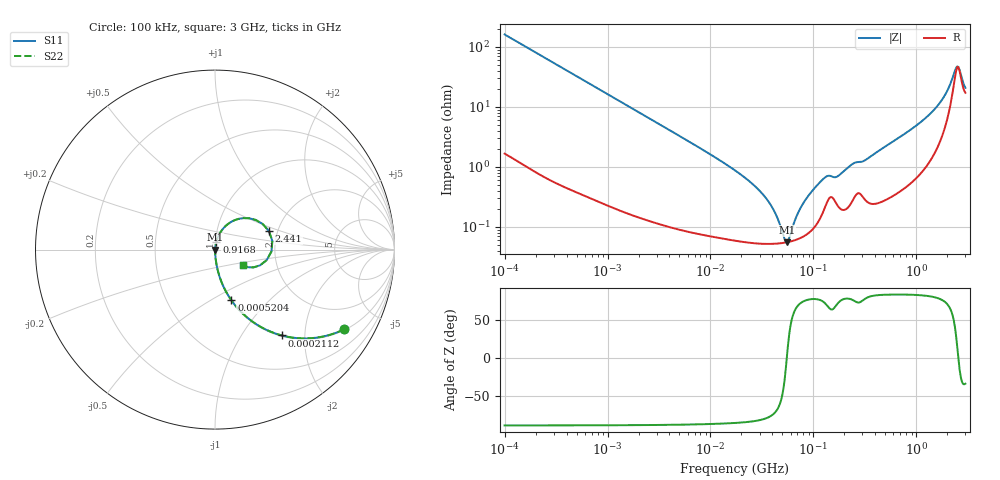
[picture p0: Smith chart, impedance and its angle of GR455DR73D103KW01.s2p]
!Murata Part Number: GR455DR73D103KW01
!These Parameters are Measured in Series Mode Connection
!Data Generated on Mar 13, 2026
!  o--ll--o
!Port1  Port2
!  o------o
!Operation Temp=25[degC], DC Bias Voltage=0[V]
!Freq. Start=100[kHz] Stop=3[GHz] 401[Steps]
# Hz S RI R 50
!Freq.(Hz) S11(Real) S11(Imag) S21(Real) S21(Imag) S12(Real) S12(Imag) S22(Real) S22(Imag)
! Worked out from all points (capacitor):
!   401 points, 100 kHz to 3 GHz, reference 50 ohm
!   read as one part in series: C = 9.88 nF near 105.3 kHz
!   lowest |Z| = 55.4 mohm at 55.24 MHz (marker M1)
!   series resonance near 55.22 MHz, so ESL is about 840 pH
!   S11 on the Smith chart (normalised r, x): 100 kHz: 1.03, -3.22; 211.2 kHz: 1.02, -1.53; 520.4 kHz: 1.01, -0.62; 916.8 MHz: 1.01, +0.09; 2.441 GHz: 1.80, +0.41; 3 GHz: 1.34, -0.23
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100000  0.7191 -0.4443  0.2809 0.4443  0.2809 0.4443  0.7191 -0.4443
211150  0.3707 -0.478  0.6293 0.478  0.6293 0.478  0.3707 -0.478
520403  0.0915 -0.2825  0.9085 0.2825  0.9085 0.2825  0.0915 -0.2825
562235  0.0798 -0.265  0.9202 0.265  0.9202 0.265  0.0798 -0.265
3161081  0.00379 -0.0516  0.9962 0.0516  0.9962 0.0516  0.00379 -0.0516
1.77727e7  0.000656 -0.00845  0.9993 0.00845  0.9993 0.00845  0.000656 -0.00845
3.564176e7  0.000528 -0.00277  0.9995 0.00277  0.9995 0.00277  0.000528 -0.00277
4.268829e7  0.000527 -0.0016  0.9995 0.0016  0.9995 0.0016  0.000527 -0.0016
5.246276e7  0.000545 -0.000317  0.9995 0.000317  0.9995 0.000317  0.000545 -0.000317
5.523785e7  0.000554 2.3e-06  0.9994 -2.3e-06  0.9994 -2.3e-06  0.000554 2.3e-06
7.334282e7  0.000645 0.00181  0.9994 -0.00181  0.9994 -0.00181  0.000645 0.00181
9.738194e7  0.00091 0.00386  0.9991 -0.00386  0.9991 -0.00386  0.00091 0.00386
1.326759e8  0.00237 0.00641  0.9976 -0.00641  0.9976 -0.00641  0.00237 0.00641
1.716802e8  0.00231 0.00654  0.9977 -0.00654  0.9977 -0.00654  0.00231 0.00654
2.400085e8  0.00283 0.0108  0.9972 -0.0108  0.9972 -0.0108  0.00283 0.0108
5.475153e8  0.00358 0.0238  0.9964 -0.0238  0.9964 -0.0238  0.00358 0.0238
9.167529e8  0.00745 0.0428  0.9926 -0.0428  0.9926 -0.0428  0.00745 0.0428
1.838476e9  0.0534 0.1259  0.9466 -0.1259  0.9466 -0.1259  0.0534 0.1259
2.201951e9  0.1571 0.1754  0.8429 -0.1754  0.8429 -0.1754  0.1571 0.1754
2.441062e9  0.3004 0.1031  0.6996 -0.1031  0.6996 -0.1031  0.3004 0.1031
2.706139e9  0.2511 -0.0875  0.7489 0.0875  0.7489 0.0875  0.2511 -0.0875
3e9  0.1549 -0.0847  0.8451 0.0847  0.8451 0.0847  0.1549 -0.0847
